TYPE UDT 1
AUTHOR : RAmann
FAMILY : KP
NAME : KPID
VERSION : 1.0


  STRUCT
   B_FC : BYTE ;	//familiy code
   B_ID1 : BYTE ;	//ID byte 1
   B_ID2 : BYTE ;	//ID byte 2
   B_ID3 : BYTE ;	//ID byte 3
   B_ID4 : BYTE ;	//ID byte 4
   B_ID5 : BYTE ;	//ID byte 5
   B_ID6 : BYTE ;	//ID byte 6
   B_CRC : BYTE ;	//CRC byte
  END_STRUCT ;
END_TYPE

TYPE UDT 2
AUTHOR : RAmann
FAMILY : KP
NAME : KPUSER
VERSION : 1.0


  STRUCT
   I_AccessLevel : INT ;	//rights of user
   I_UserID : INT ;	//user identification number
   TXT_UserData : STRING  [94 ];	//user name
  END_STRUCT ;
END_TYPE

DATA_BLOCK DB 2
TITLE =
AUTHOR : RAmann
FAMILY : KP
NAME : KPUSRLST
VERSION : 1.0


  STRUCT
   UDT_ActualUser : UDT 2;	//user data corresponding to found key
   AS_KeyList : ARRAY  [1 .. 4 ] OF STRUCT
    UDT_Key : UDT 1;	//ID of key
    UDT_User : UDT 2;	//data of corresponding user
   END_STRUCT ;
  END_STRUCT ;
BEGIN
   UDT_ActualUser.I_AccessLevel := 0;
   UDT_ActualUser.I_UserID := 0;
   UDT_ActualUser.TXT_UserData := '';
   AS_KeyList[1].UDT_Key.B_FC := B#16#1;
   AS_KeyList[1].UDT_Key.B_ID1 := B#16#D5;
   AS_KeyList[1].UDT_Key.B_ID2 := B#16#2F;
   AS_KeyList[1].UDT_Key.B_ID3 := B#16#BF;
   AS_KeyList[1].UDT_Key.B_ID4 := B#16#C;
   AS_KeyList[1].UDT_Key.B_ID5 := B#16#0;
   AS_KeyList[1].UDT_Key.B_ID6 := B#16#0;
   AS_KeyList[1].UDT_Key.B_CRC := B#16#35;
   AS_KeyList[1].UDT_User.I_AccessLevel := 1;
   AS_KeyList[1].UDT_User.I_UserID := 100;
   AS_KeyList[1].UDT_User.TXT_UserData := 'Testuser 1';
   AS_KeyList[2].UDT_Key.B_FC := B#16#0;
   AS_KeyList[2].UDT_Key.B_ID1 := B#16#0;
   AS_KeyList[2].UDT_Key.B_ID2 := B#16#0;
   AS_KeyList[2].UDT_Key.B_ID3 := B#16#0;
   AS_KeyList[2].UDT_Key.B_ID4 := B#16#0;
   AS_KeyList[2].UDT_Key.B_ID5 := B#16#0;
   AS_KeyList[2].UDT_Key.B_ID6 := B#16#0;
   AS_KeyList[2].UDT_Key.B_CRC := B#16#0;
   AS_KeyList[2].UDT_User.I_AccessLevel := 0;
   AS_KeyList[2].UDT_User.I_UserID := 0;
   AS_KeyList[2].UDT_User.TXT_UserData := '';
   AS_KeyList[3].UDT_Key.B_FC := B#16#0;
   AS_KeyList[3].UDT_Key.B_ID1 := B#16#0;
   AS_KeyList[3].UDT_Key.B_ID2 := B#16#0;
   AS_KeyList[3].UDT_Key.B_ID3 := B#16#0;
   AS_KeyList[3].UDT_Key.B_ID4 := B#16#0;
   AS_KeyList[3].UDT_Key.B_ID5 := B#16#0;
   AS_KeyList[3].UDT_Key.B_ID6 := B#16#0;
   AS_KeyList[3].UDT_Key.B_CRC := B#16#0;
   AS_KeyList[3].UDT_User.I_AccessLevel := 0;
   AS_KeyList[3].UDT_User.I_UserID := 0;
   AS_KeyList[3].UDT_User.TXT_UserData := '';
   AS_KeyList[4].UDT_Key.B_FC := B#16#0;
   AS_KeyList[4].UDT_Key.B_ID1 := B#16#0;
   AS_KeyList[4].UDT_Key.B_ID2 := B#16#0;
   AS_KeyList[4].UDT_Key.B_ID3 := B#16#0;
   AS_KeyList[4].UDT_Key.B_ID4 := B#16#0;
   AS_KeyList[4].UDT_Key.B_ID5 := B#16#0;
   AS_KeyList[4].UDT_Key.B_ID6 := B#16#0;
   AS_KeyList[4].UDT_Key.B_CRC := B#16#0;
   AS_KeyList[4].UDT_User.I_AccessLevel := 0;
   AS_KeyList[4].UDT_User.I_UserID := 0;
   AS_KeyList[4].UDT_User.TXT_UserData := '';
END_DATA_BLOCK

FUNCTION_BLOCK FB 1
TITLE =Read Key-ID and find corresponding user data
//IANYw_ActualUser
//----------------
//The FB fills the memory area addressed by this pointer with the user data
//corresponding with actually applied key. The length of the memory area is used
//to estimate the number of datasets addressed by IANYr_KeyList.
//
//IANYr_KeyList
//-------------
//This pointer must refer to a list of datasets, where each dataset consists of a
//key-ID and the corresponding user data. Length of the key-ID is 8 byte. Length
//of the user data must be equal to the length of the area addressed by
//IANYw_ActualUser.
//Example:
//
//addresses by IANYr_KeyList:
//   AS_KeyList : ARRAY  [1 .. 4 ] OF STRUCT //list of four datasets
//    S_Key : STRUCT //KEY-ID
//     B_FC : BYTE ;// familiy code
//     B_ID1 : BYTE ;// ID byte 1
//     B_ID2 : BYTE ;// ID byte 2
//     B_ID3 : BYTE ;// ID byte 3
//     B_ID4 : BYTE ;// ID byte 4
//     B_ID5 : BYTE ;// ID byte 5
//     B_ID6 : BYTE ;// ID byte 6
//     B_CRC : BYTE ;// CRC byte
//    END_STRUCT ;
//    S_User : STRUCT //USER DATA
//     I_AccessLevel : INT ;// rights of user
//     I_UserID : INT ;// user identification number
//     TXT_UserData : STRING  [94 ];// user name
//    END_STRUCT ;
//   END_STRUCT ;
//
//addressed by IANYw_ActualUser:
//   S_ActualUser : STRUCT //USER DATA
//    I_AccessLevel : INT ;// rights of user
//    I_UserID : INT ;// user identification number
//    TXT_UserData : STRING  [94 ];// user name
//   END_STRUCT ;
AUTHOR : RAmann
FAMILY : KP
NAME : KPCHKUSR
VERSION : 1.0


VAR_INPUT
  IANYw_ActualUser : ANY ;	//pointer on buffer for actual user data [length 1*UDT2; write]
  IANYr_KeyList : ANY ;	//pointer on table with known keys and user data [length N*(UDT1+UDT2); read]
  II_StartAddressIn : INT ;	//input start address of KeyPilot (according to HW-Config)
END_VAR
VAR
  SADW_KeyID : ARRAY  [1 .. 2 ] OF //buffer for key-id
  DWORD ;
  SDW_EntryAddress : DWORD ;	//start address of found entry
  SI_RetVal : INT ;	//state information of SFC14 "DPRD_DAT"
  SI_DataNumber : INT ;	//numer of keys in table
  SI_LoopCounter : INT ;	//loop counter
  SI_UserDataSize : INT ;	//size of user data
  SI_KeyDataSize : INT ;	//size of key data (id + user data)
  SI_EntryNumber : INT ;	//number of found entry in list of known keys
  SI_LastEntryNumber : INT ;	//number of found entry at last cycle
  SW_StartAddressIn : WORD ;	//input start address from HW-Config
  S_KeyApplied : BOOL ;	//flag is true if a key is applied to the KeyPilot reading head
END_VAR
VAR_TEMP
  LANYr_FoundUser : ANY ;	//pointer to user data corresponding with found key
  LANYw_ActualUser : ANY ;	//pointer to user data corresponding with found key
  LDW_AR1 : DWORD ;	//buffer for address register 1
  LDW_AR2 : DWORD ;	//buffer for address register 2
  LW_DB : WORD ;	//number of DB with key table
END_VAR
BEGIN
NETWORK
TITLE =backup of address register

      TAR1  #LDW_AR1;
      TAR2  #LDW_AR2;

NETWORK
TITLE =clear values

      L     #SI_EntryNumber;
      T     #SI_LastEntryNumber;

      L     0;
      T     #SI_EntryNumber;

NETWORK
TITLE =read key id

      L     #II_StartAddressIn; // type cast from INT to WORD
      T     #SW_StartAddressIn;

      CALL SFC   14 (// read data from KeyPilot
           LADDR                    := #SW_StartAddressIn,
           RET_VAL                  := #SI_RetVal,
           RECORD                   := #SADW_KeyID);

NETWORK
TITLE =check pointer to buffer for actual user

// get address of pointer
      L     P##IANYw_ActualUser;
      LAR1  ;

// check data type
      L     B [AR1,P#1.0]; // data type stored in ANY-pointer
      L     2;
      <>I   ;
      SPB   mend; // jump if data type is not BYTE

// get length of data area
      L     W [AR1,P#2.0]; // repeat counter (area length) stored in ANY-pointer
      T     #SI_UserDataSize;
      L     8; // size of key-id
      +I    ;
      T     #SI_KeyDataSize;

NETWORK
TITLE =check pointer to data table

// get address of pointer
      L     P##IANYr_KeyList;
      LAR1  ;

// check data type
      L     B [AR1,P#1.0]; // data type stored in ANY-pointer
      L     2;
      <>I   ;
      SPB   mend; // jump if data type is not BYTE

// check length of data area
      L     W [AR1,P#2.0]; // repeat counter (area length) stored in ANY-pointer
      L     #SI_KeyDataSize;
      /I    ;
      T     #SI_DataNumber; // store integral result of division
      SRD   16; // move remainder to the right
      L     0;
      <>I   ;
      SPB   mend; // jump if length of data area is not a multiple of key-data size

// open DB
      L     0;
      L     W [AR1,P#4.0]; // number of DB stored in ANY-pointer
      ==I   ;
      SPB   mdb1; // jump if data area is not part of a DB
      T     #LW_DB;
      AUF   DB [#LW_DB];

// get address of data area
mdb1: L     D [AR1,P#6.0]; // Adresse im ANY-Zeiger
      LAR1  ;

NETWORK
TITLE =key applied?

      O(    ;
      L     #SADW_KeyID[1];
      L     0;
      <>D   ;
      )     ;
      O(    ;
      L     #SADW_KeyID[2];
      L     0;
      <>D   ;
      )     ;
      =     #S_KeyApplied;
      SPBN  mnot; // jump if no key is applied to reading head

NETWORK
TITLE =search loop

      L     #SI_DataNumber;
mnxt: T     #SI_LoopCounter;

      U(    ;
      L     #SADW_KeyID[1];
      L     D [AR1,P#0.0]; // key-id from data area, part 1
      ==D   ;
      )     ;
      U(    ;
      L     #SADW_KeyID[2];
      L     D [AR1,P#4.0]; // key-id from data area, part 2
      ==D   ;
      )     ;
      SPB   mok;

      L     #SI_KeyDataSize;
      SLW   3;
      +AR1  ; // get address of next key-data in data area

      L     #SI_LoopCounter;
      LOOP  mnxt;
      SPA   mnot;

mok:  TAR1  ;
      T     #SDW_EntryAddress; // store start address of found entry

      L     #SI_DataNumber;
      L     #SI_LoopCounter;
      -I    ;
      L     1;
      +I    ;
      T     #SI_EntryNumber;

NETWORK
TITLE =enable copying of user data

mnot: L     #SI_EntryNumber;
      L     #SI_LastEntryNumber;
      ==I   ;
      SPB   mend;

NETWORK
TITLE =create source pointer

// get address of pointer
      L     P##LANYr_FoundUser;
      LAR1  ;
      L     P##IANYr_KeyList;
      LAR2  ;

// copy data type
      L     W [AR2,P#0.0]; // part of pointer IANYr_KeyList
      T     W [AR1,P#0.0]; // part of pointer LANYr_FoundUser

// copy DB number
      L     W [AR2,P#4.0];
      T     W [AR1,P#4.0];

// restore AR2
      LAR2  #LDW_AR2;

// write data length
      L     #SI_UserDataSize;
      T     W [AR1,P#2.0];

// write address
      L     8; // size of key-id
      SLW   3;
      L     #SDW_EntryAddress;
      +D    ;
      T     D [AR1,P#6.0];

NETWORK
TITLE =create destination pointer

// get address of pointer
      L     P##LANYw_ActualUser;
      LAR1  ;
      L     P##IANYw_ActualUser;
      LAR2  ;

// copy pointer information
      L     D [AR2,P#0.0]; // part of pointer IANYw_ActualUser
      T     D [AR1,P#0.0]; // part of pointer LANYw_ActualUser
      L     D [AR2,P#4.0];
      T     D [AR1,P#4.0];
      L     W [AR2,P#8.0];
      T     W [AR1,P#8.0];

// restore AR2
      LAR2  #LDW_AR2;

NETWORK
TITLE =copy/clear user data

      U     #S_KeyApplied;
      SPBN  mclr;

      CALL SFC   20 (
           SRCBLK                   := #LANYr_FoundUser,
           RET_VAL                  := #SI_RetVal,
           DSTBLK                   := #LANYw_ActualUser);

      SPA   mend;

mclr: CALL SFC   21 (
           BVAL                     := #SI_EntryNumber,// if function is called, entry number is zero -> empty fill pattern
           RET_VAL                  := #SI_RetVal,
           BLK                      := #LANYw_ActualUser);

NETWORK
TITLE =restore address register

mend: LAR1  #LDW_AR1;
      LAR2  #LDW_AR2;

END_FUNCTION_BLOCK

DATA_BLOCK DB 3
TITLE =
AUTHOR : RAmann
FAMILY : KP
VERSION : 0.0

 FB 1
BEGIN
   II_StartAddressIn := 0;
   SADW_KeyID[1] := DW#16#0;
   SADW_KeyID[2] := DW#16#0;
   SDW_EntryAddress := DW#16#0;
   SI_RetVal := 0;
   SI_DataNumber := 0;
   SI_LoopCounter := 0;
   SI_UserDataSize := 0;
   SI_KeyDataSize := 0;
   SI_EntryNumber := 0;
   SI_LastEntryNumber := 0;
   SW_StartAddressIn := W#16#0;
   S_KeyApplied := FALSE;
END_DATA_BLOCK

ORGANIZATION_BLOCK OB 1
TITLE = "Main Program Sweep (Cycle)"
//3. User Data
//------------
//
//In this example the actual key at the KeyPilot is searched in a database of
//known keys. If the key matches with a database entry, the program copies the
//user data stored with the database entry to a buffer for actual user data. The
//LED is controlled depending on the "access-level" in this buffer.
//
//For testing you have to adapt the database (DB2, array AS_KeyList) by
//inserting the key-IDs you want to search for and the user data according to the
//keys (e.g. in data view). Create user data with entry "I_AccesLevel" higher
//than 0.
//
//There are two UDTs:
//UDT1 ("KeyPilot_Id") is used for key-IDs an has a size of 8 byte.
//UDT2 ("KeyPilot_UserData") is used for the user data. You may change the
//structure and size of it to your needs. FB1 ("KeyPilot_CheckUser") doesn't care
//about the content of the user data. FB1 derives the offset in DB2.AS_KeyList
//between the different key-IDs from the size of DB1.UDT_ActualUser. Make sure to
//preserve this relation and to set the pointers to the key list and the actual
//user buffer correctly.
AUTHOR : RAmann
FAMILY : KP
NAME : KPMAIN
VERSION : 1.0


VAR_TEMP
  OB1_EV_CLASS : BYTE ;	//Bits 0-3 = 1 (Coming event), Bits 4-7 = 1 (Event class 1)
  OB1_SCAN_1 : BYTE ;	//1 (Cold restart scan 1 of OB 1), 3 (Scan 2-n of OB 1)
  OB1_PRIORITY : BYTE ;	//Priority of OB Execution
  OB1_OB_NUMBR : BYTE ;	//1 (Organization block 1, OB1)
  OB1_RESERVED_1 : BYTE ;	//Reserved for system
  OB1_RESERVED_2 : BYTE ;	//Reserved for system
  OB1_PREV_CYCLE : INT ;	//Cycle time of previous OB1 scan (milliseconds)
  OB1_MIN_CYCLE : INT ;	//Minimum cycle time of OB1 (milliseconds)
  OB1_MAX_CYCLE : INT ;	//Maximum cycle time of OB1 (milliseconds)
  OB1_DATE_TIME : DATE_AND_TIME ;	//Date and time OB1 started
END_VAR
BEGIN
NETWORK
TITLE =read key-ID and check database

      CALL FB     1 , DB     3 (
           IANYw_ActualUser         := DB2.UDT_ActualUser,
           IANYr_KeyList            := DB2.AS_KeyList,
           II_StartAddressIn        := 10);

NETWORK
TITLE =control LED

// LED control: set LED to green if access level is greater than zero
      L     DB2.DBW    0;
      L     0;
      >I    ;
      =     A     10.1;
      NOT   ;
      =     A     10.0;

END_ORGANIZATION_BLOCK

